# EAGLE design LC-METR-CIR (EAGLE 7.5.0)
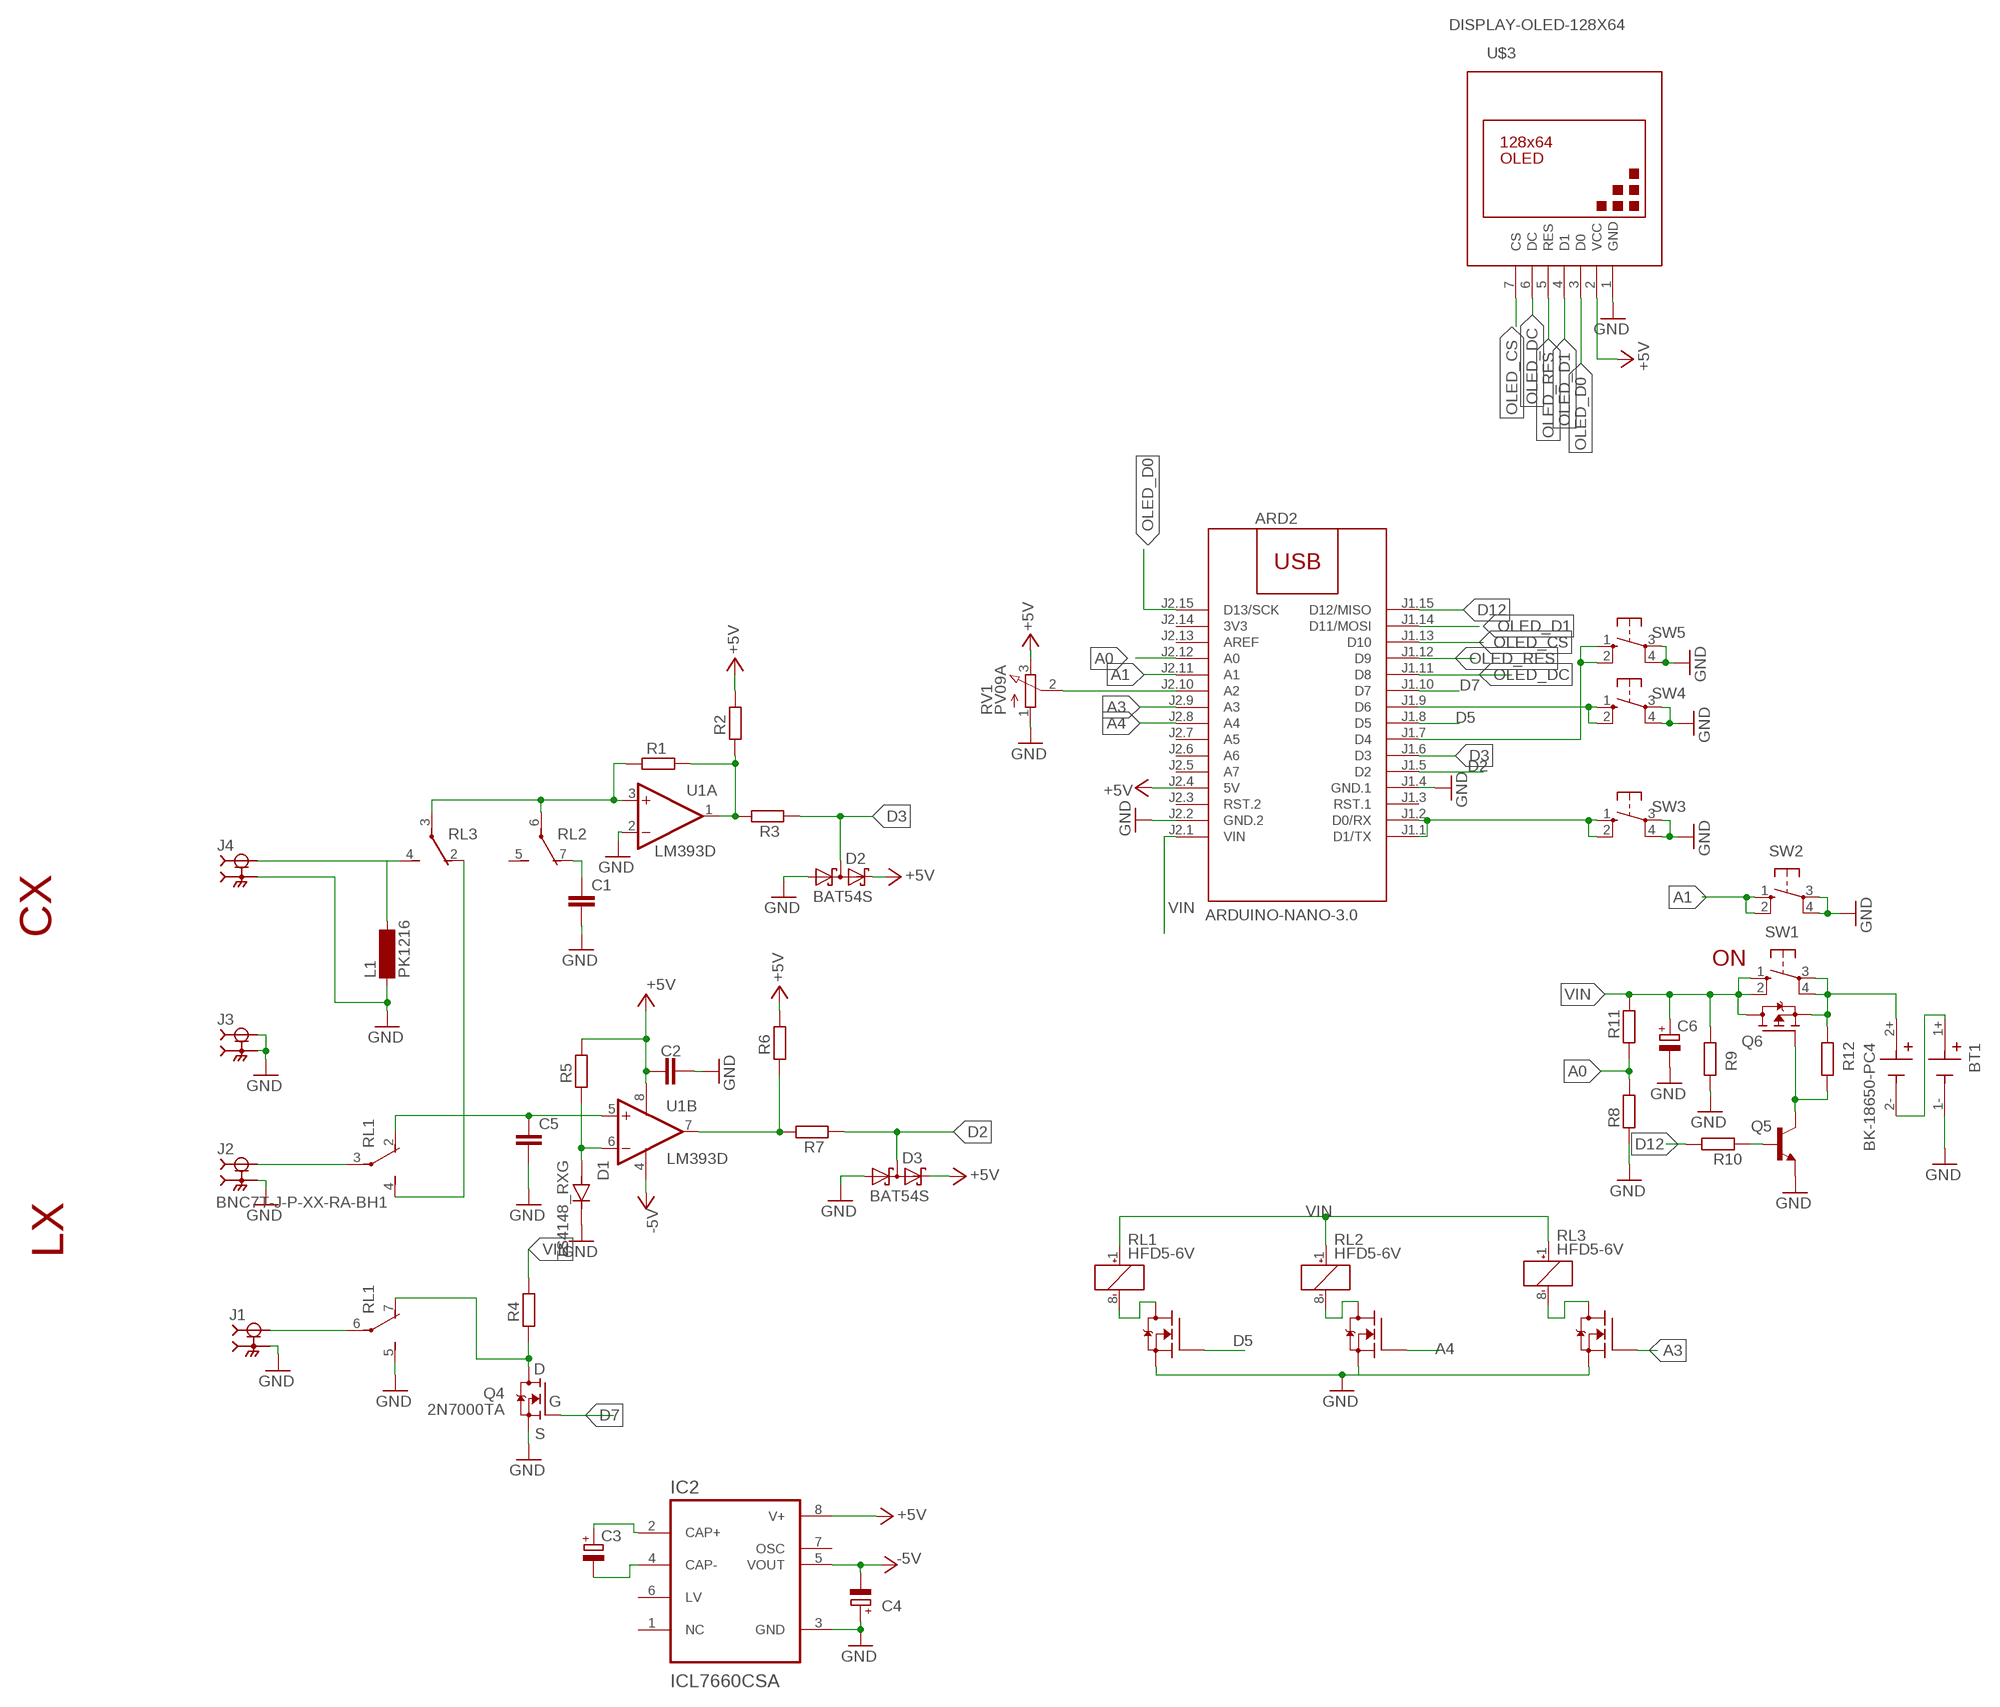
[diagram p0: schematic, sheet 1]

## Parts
ARD2  ARDUINO-NANO-3.0  [ARDUINO-NANO-3.0]
BT1  BK-18650-PC4  [BAT_BK-18650-PC4]
C1  C-EUC1206  [C1206]
C2  C-EUC0805  [C0805]
C3  CPOL-EUSMCA  [SMC_A]
C4  CPOL-EUSMCA  [SMC_A]
C5  C-EUC1206  [C1206]
C6  CPOL-EUSMCA  [SMC_A]
D1  TS4148_RXG  [DIO_TS4148_RXG]
D2  BAT54S  [SOT23]
D3  BAT54S  [SOT23]
IC2  ICL7660CSA  [SOIC127P600X175-8N]
J1  BNC7T-J-P-XX-RA-BH1  [SAMTEC_BNC7T-J-P-XX-RA-BH1]
J2  BNC7T-J-P-XX-RA-BH1  [SAMTEC_BNC7T-J-P-XX-RA-BH1]
J3  BNC7T-J-P-XX-RA-BH1  [SAMTEC_BNC7T-J-P-XX-RA-BH1]
J4  BNC7T-J-P-XX-RA-BH1  [SAMTEC_BNC7T-J-P-XX-RA-BH1]
L1  PK1216  BS11  [BS11]
Q1  ZVN3310F  [SOT23]
Q2  ZVN3310F  [SOT23]
Q3  ZVN3310F  [SOT23]
Q4  2N7000TA  [TO-92]
Q5  BC817-16LT1SMD  [SOT23-BEC]
Q6  STR2P3LLH6  [SOT23]
R1  R-EU_R0805  [R0805]
R2  R-EU_R0805  [R0805]
R3  R-EU_R0805  [R0805]
R4  R-EU_R0805  [R0805]
R5  R-EU_R0805  [R0805]
R6  R-EU_R0805  [R0805]
R7  R-EU_R0805  [R0805]
R8  R-EU_R0805  [R0805]
R9  R-EU_R0805  [R0805]
R10  R-EU_R0805  [R0805]
R11  R-EU_R0805  [R0805]
R12  R-EU_R0805  [R0805]
RL1  HFD5-6V  G6J-2P-Y  [G6J-2P-Y]
RL2  HFD5-6V  G6J-2P-Y  [G6J-2P-Y]
RL3  HFD5-6V  G6J-2P-Y  [G6J-2P-Y]
RV1  PV09A  [PTV09]
SW1  10-XX  [B3F-10XX]
SW2  10-XX  [B3F-10XX]
SW3  10-XX  [B3F-10XX]
SW4  10-XX  [B3F-10XX]
SW5  10-XX  [B3F-10XX]
U1  LM393D  [SO08]
U$3  DISPLAY-OLED-128X64  [DISPLAY-OLED-128X64]

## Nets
+5V: ARD2.J2.4(5V) C2.1 D2.2(C2) D3.2(C2) IC2.8(V+) R2.2 R5.2 R6.2 RV1.3(E) U1.8(P:V+) U$3.2(VCC)
-5V: C4.- IC2.5(VOUT) U1.4(P:V-)
A0: ARD2.J2.12(A0) R8.2 R11.1
A1: ARD2.J2.11(A1) SW2.1(S) SW2.2(S1)
A3: ARD2.J2.9(A3) Q1.2(G)
A4: ARD2.J2.8(A4) Q2.2(G)
BAT: BT1.2+ Q6.3(S) R12.2 SW1.3(P) SW1.4(P1)
D2: ARD2.J1.5(D2) D3.3(C1A2) R7.1
D3: ARD2.J1.6(D3) D2.3(C1A2) R3.1
D5: ARD2.J1.8(D5) Q3.2(G)
D7: ARD2.J1.10(D7) Q4.2(G)
D12: ARD2.J1.15(D12/MISO) R10.2
GND: ARD2.J1.4(GND.1) ARD2.J2.2(GND.2) BT1.1- C1.2 C2.2 C4.+ C5.2 C6.- D1.C(K) D2.1(A1) D3.1(A1) IC2.3(GND) J1.S1 J1.S2 J1.S3 J1.S4 J2.S1 J2.S2 J2.S3 J2.S4 J3.1 J3.S1 J3.S2 J3.S3 J3.S4 J4.S1 J4.S2 J4.S3 J4.S4 L1.1 Q1.3(S) Q2.3(S) Q3.3(S) Q4.1(S) Q5.E R8.1 R9.1 RL1.5(3:S) RV1.1(A) SW2.3(P) SW2.4(P1) SW3.3(P) SW3.4(P1) SW4.3(P) SW4.4(P1) SW5.3(P) SW5.4(P1) U1.2(A:-IN) U$3.1(GND)
N$1: ARD2.J1.1(D1/TX) ARD2.J1.2(D0/RX) SW3.1(S) SW3.2(S1)
N$2: ARD2.J1.9(D6) SW4.1(S) SW4.2(S1)
N$3: R1.1 RL2.6(3:P) RL3.3(2:P) U1.3(A:+IN)
N$4: R1.2 R2.1 R3.2 U1.1(A:OUT)
N$5: ARD2.J1.7(D4) SW5.1(S) SW5.2(S1)
N$6: C3.+ IC2.2(CAP+)
N$7: ARD2.J2.10(A2) RV1.2(S)
N$8: C3.- IC2.4(CAP-)
N$9: R6.1 R7.2 U1.7(B:OUT)
N$10: C1.1 RL2.7(3:O)
N$11: J4.1 L1.2 RL3.4(2:S)
N$12: C5.1 RL1.2(2:O) U1.5(B:+IN)
N$13: RL1.4(2:S) RL3.2(2:O)
N$14: Q4.3(D) R4.1 RL1.7(3:O)
N$15: J2.1 RL1.3(2:P)
N$16: Q5.C Q6.2(G) R12.1
N$17: J1.1 RL1.6(3:P)
N$18: Q5.B R10.1
N$19: Q3.1(D) RL1.8(1:-)
N$20: Q2.1(D) RL2.8(1:-)
N$21: Q1.1(D) RL3.8(1:-)
N$22: BT1.1+ BT1.2-
N$23: D1.A R5.1 U1.6(B:-IN)
OLED_CS: ARD2.J1.13(D10) U$3.7(CS)
OLED_D0: ARD2.J2.15(D13/SCK) U$3.3(D0)
OLED_D1: ARD2.J1.14(D11/MOSI) U$3.4(D1)
OLED_DC: ARD2.J1.11(D8) U$3.6(DC)
OLED_RES: ARD2.J1.12(D9) U$3.5(RES)
VIN: ARD2.J2.1(VIN) C6.+ Q6.1(D) R4.2 R9.2 R11.2 RL1.1(1:+) RL2.1(1:+) RL3.1(1:+) SW1.1(S) SW1.2(S1)
Unconnected: ARD2.J1.3(RST.1) ARD2.J2.3(RST.2) ARD2.J2.5(A7) ARD2.J2.6(A6) ARD2.J2.7(A5) ARD2.J2.13(AREF) IC2.1(NC) IC2.6(LV) IC2.7(OSC) RL2.2(2:O) RL2.3(2:P) RL2.4(2:S) RL2.5(3:S) RL3.5(3:S) RL3.6(3:P) RL3.7(3:O)

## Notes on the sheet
- CX
- ON
- LX

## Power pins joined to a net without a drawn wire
3V3: ARD2.J2.14(3V3)

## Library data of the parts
ARD2 = diy-modules:ARDUINO-NANO-3.0: Arduino Nano 3.0 and compatible devices More details available here: https://www.arduino.cc/en/Main/ArduinoBoardNano Click here to find device on ebay.com
BT1 = BK-18650-PC4:BK-18650-PC4: Battery Holder (Open) 18650 2 Cell PC Pin Check availability; AVAILABILITY: In Stock; CHECK_PRICES: https://www.snapeda.com/parts/BK-18650-PC4/Memory+Protection+Devices/view-part/?ref=eda; DESCRIPTION: Battery Holder (Open) 18650 2 Cell PC Pin; MF: MPD (Memory Protection Devices); MP: BK-18650-PC4; PACKAGE: None; PRICE: None; SNAPEDA_LINK: https://www.snapeda.com/parts/BK-18650-PC4/Memory+Protection+Devices/view-part/?ref=snap
C1 C2 C5 = rcl:C-EU: CAPACITOR, European symbol
C3 C4 C6 = rcl:CPOL-EU: POLARIZED CAPACITOR, European symbol
D1 = TS4148_RXG:TS4148_RXG: Check availability Check availability Check availability; AVAILABILITY: In Stock; CHECK_PRICES: https://www.snapeda.com/parts/TS4148%20RXG/Taiwan+Semiconductor/view-part/?ref=eda; DESCRIPTION: 1206 (Ceramics) 75V 0.15A Switching Diode & Array; MF: Taiwan Semiconductor; MP: TS4148 RXG; PACKAGE: 1206-2 Taiwan Semiconductor; PRICE: None; SNAPEDA_LINK: https://www.snapeda.com/parts/TS4148%20RXG/Taiwan+Semiconductor/view-part/?ref=snap
D2 D3 = diode:BAT54S: Schottky Diodes Pin connection corrected 2011-05-04 Source: Fairchild .. BAT54.pdf
IC2 = ICL7660CSA:ICL7660CSA: Check availability; AVAILABILITY: In Stock; CHECK_PRICES: https://www.snapeda.com/parts/ICL7660CSA/Analog+Devices/view-part/?ref=eda; DESCRIPTION: Charge Pump Switching Regulator IC Positive or Negative Fixed -Vin, nVin, Vin/2 1 Output 20mA 8-SOIC (0.154, 3.90mm Width); MF: Analog Devices; MP: ICL7660CSA; PACKAGE: SOIC-8 Maxim; PRICE: None; SNAPEDA_LINK: https://www.snapeda.com/parts/ICL7660CSA/Analog+Devices/view-part/?ref=snap
J1-J4 = BNC7T-J-P-XX-RA-BH1:BNC7T-J-P-XX-RA-BH1: TRUE 75 OHM RIGHT ANGLE JACK ASSEMBLY Check availability; AVAILABILITY: In Stock; CHECK_PRICES: https://www.snapeda.com/parts/BNC7T-J-P-HN-RA-BH1/Samtec+Inc./view-part/?ref=eda; DESCRIPTION: BNC Connector Jack, Female Socket 75 Ohms Panel Mount, Through Hole, Right Angle Solder; MF: Samtec; MP: BNC7T-J-P-HN-RA-BH1; PACKAGE: None; PRICE: None; PURCHASE-URL: https://www.snapeda.com/api/url_track_click_mouser/?unipart_id=608953&manufacturer=Samtec&part_name=BNC7T-J-P-HN-RA-BH1&search_term=bnc connector; SNAPEDA_LINK: https://www.snapeda.com/parts/BNC7T-J-P-HN-RA-BH1/Samtec+Inc./view-part/?ref=snap
L1 = inductor-neosid:BS: INDUCTOR; OC_FARNELL: unknown; OC_NEWARK: unknown
Q1-Q3 = transistor-fet:ZVN3310F
Q4 = 2N7000TA:2N7000TA: http://www.mouser.com/ds/2/149/2N7000TA-347571.pdf Check availability; AVAILABILITY: In Stock; CHECK_PRICES: https://www.snapeda.com/parts/2N7000-TA/Onsemi/view-part/?ref=eda; DESCRIPTION: N-Channel 60 V 200mA (Tc) 400mW (Ta) Through Hole TO-92-3; MF: ON Semiconductor; MP: 2N7000-TA; PACKAGE: E-PKG AXIAL-LEADED-2 ON Semiconductor; PRICE: None; SNAPEDA_LINK: https://www.snapeda.com/parts/2N7000-TA/Onsemi/view-part/?ref=snap
Q5 = transistor-npn:BC817*: NPN Transistor
Q6 = transistor-fet:STR2P3LLH6
R1-R12 = rcl:R-EU_: RESISTOR, European symbol
RL1-RL3 = relay:G6J*-2?-Y: Surface-Mounting Signal Relay - G6J-Y 5.7 x 10.6 x 9 mm Source: http://www.omroncomponents.eu/ .. K125-E2-02-X.pdf; MF: OMRON COMPONENTS USA; MPN: G6J-2P-Y-DC12; OC_FARNELL: unknown; OC_NEWARK: 70J9830
RV1 = pot:PV09A
SW1-SW5 = switch-omron:10-XX: OMRON SWITCH; MPN: B3F-1000; OC_FARNELL: 176432; OC_NEWARK: 36M3542
U1 = linear:LM393: COMPARATOR
U$3 = diy-modules:DISPLAY-OLED-128X64: 128x64 Dot Matrix OLED Module based on SSD1306 chip Variant with SPI interface More details available here: http://www.instructables.com/id/How-to-use-OLED-display-arduino-module/ SSD1306 datasheet: https://cdn-shop.adafruit.com/datasheets/SSD1306.pdf Click here to find device on ebay.com Note: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

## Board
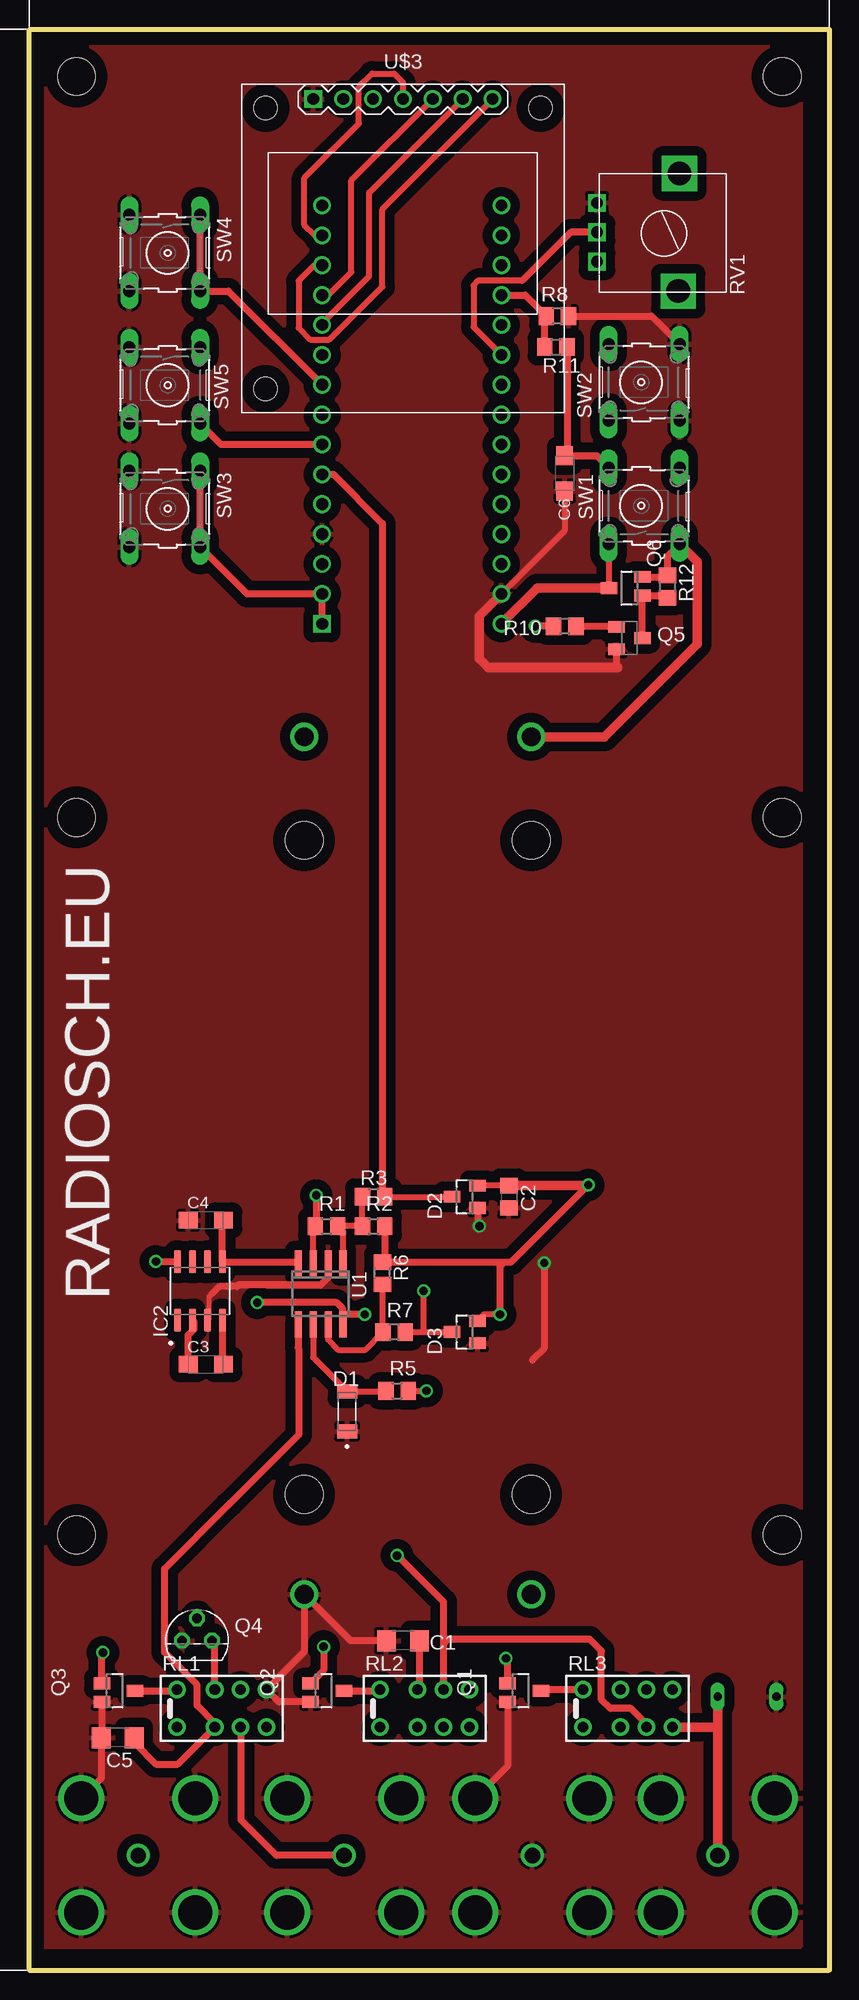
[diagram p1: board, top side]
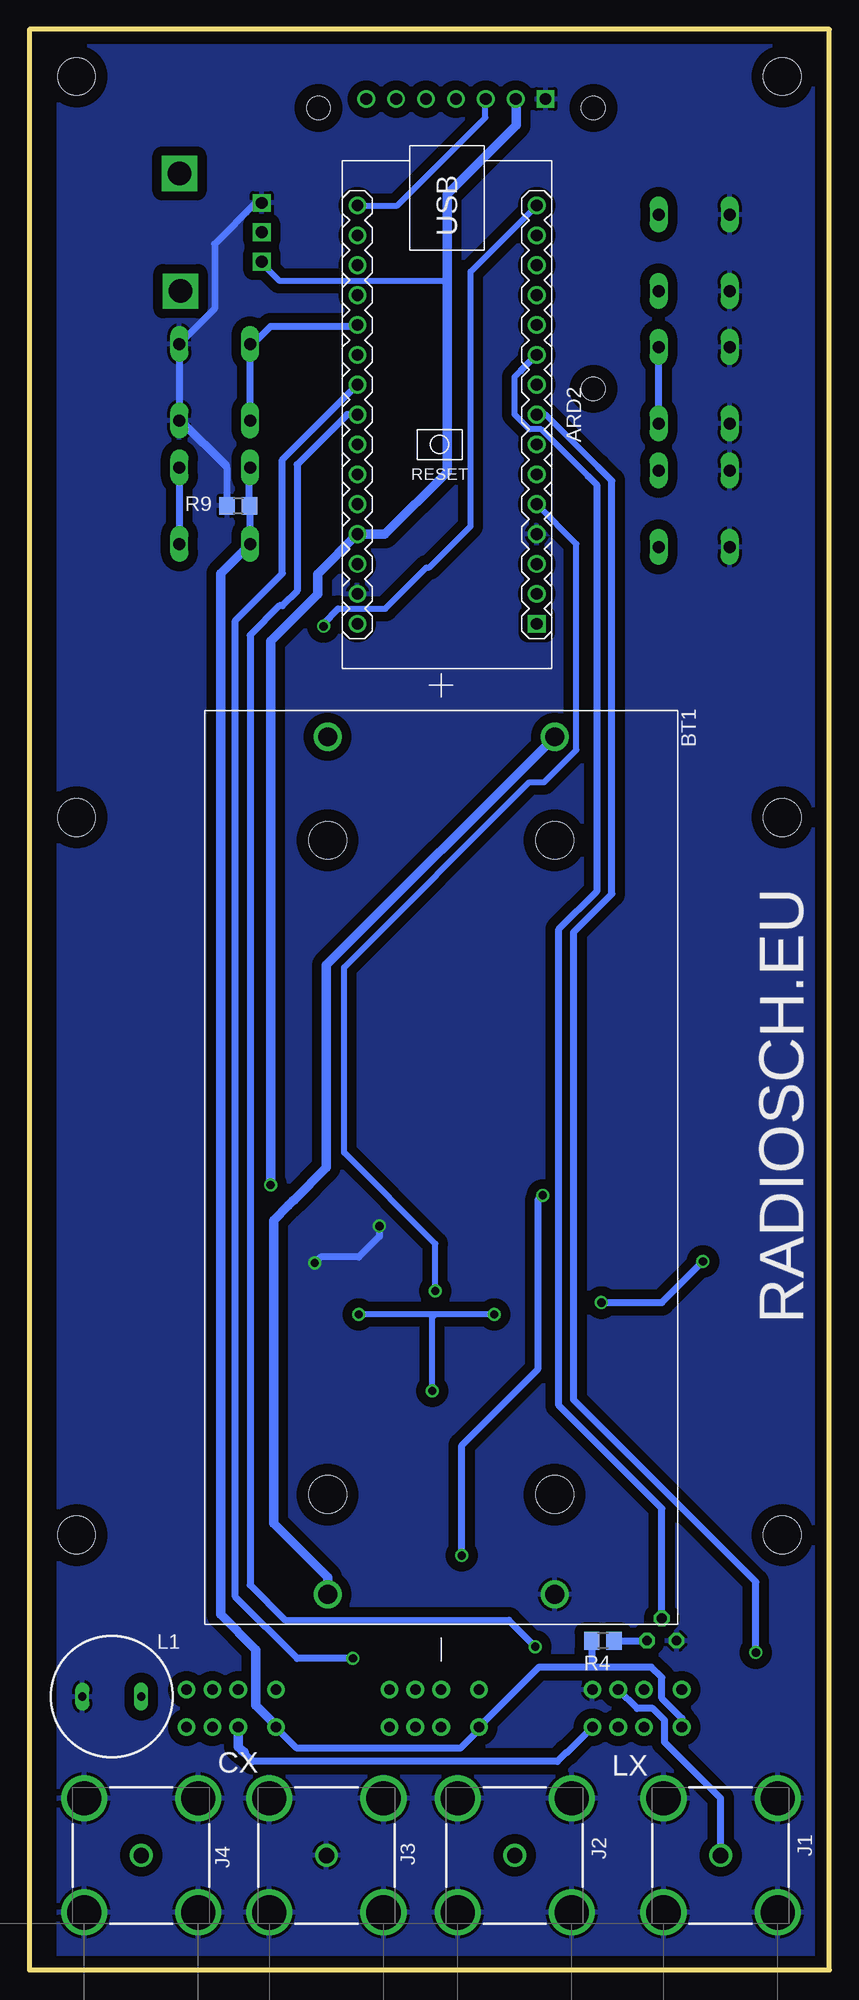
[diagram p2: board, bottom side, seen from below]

Size 68 x 165 mm. Coordinates in mm from the lower left corner, seen from the top.
Outline: 0,0 0,165 68,165 68,0 0,0
Copper layers (1*16): Top 0.035mm / dielectric 1.5mm / Bottom 0.035mm
Design rules "default *": minimum track width 10mil, minimum drill 15mil, track to track 6mil, track to pad 6mil, pad to pad 6mil, via to via 6mil, smd to smd 4mil, copper to edge 40mil, drill to drill 8mil, minimum pad ring 10mil, minimum via ring 8mil, stop-mask expansion 4mil, vias tented up to drill 0mil, thermal gap 10mil
Holes 3.2 mm at 4,161 64,161 4,98 64,98 4,37 64,37

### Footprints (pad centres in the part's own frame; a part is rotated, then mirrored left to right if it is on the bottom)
ARDUINO-NANO-3.0 = drill 1 square: J1.1 17.78,7.62 | drill 1: J1.2 15.24,7.62; J1.3 12.7,7.62; J1.4 10.16,7.62; J1.5 7.62,7.62; J1.6 5.08,7.62; J1.7 2.54,7.62; J1.8 0,7.62; J1.9 -2.54,7.62; J1.10 -5.08,7.62; J1.11 -7.62,7.62; J1.12 -10.16,7.62; J1.13 -12.7,7.62; J1.14 -15.24,7.62; J1.15 -17.78,7.62; J2.1 17.78,-7.62; J2.2 15.24,-7.62; J2.3 12.7,-7.62; J2.4 10.16,-7.62; J2.5 7.62,-7.62; J2.6 5.08,-7.62; J2.7 2.54,-7.62; J2.8 0,-7.62; J2.9 -2.54,-7.62; J2.10 -5.08,-7.62; J2.11 -7.62,-7.62; J2.12 -10.16,-7.62; J2.13 -12.7,-7.62; J2.14 -15.24,-7.62; J2.15 -17.78,-7.62
BAT_BK-18650-PC4 = drill 1.6: 1+ -36.6,9.65; 1- 36.3,9.65; 2+ -36.6,-9.65; 2- 36.3,-9.65 | hole 3.2: -27.81,-9.65; -27.81,9.65; 27.81,-9.65; 27.81,9.65
C1206 = smd 1.6 x 1.8: 1 -1.4,0; 2 1.4,0
C0805 = smd 1.3 x 1.5: 1 -0.95,0; 2 0.95,0
SMC_A = smd 1.6 x 1.4: + -1.5,0; - 1.5,0
DIO_TS4148_RXG = smd 1.2 x 1.7: A 1.7,0; C -1.7,0
SOT23 = smd 1 x 1.4: 1 -0.95,-1.1; 2 0.95,-1.1; 3 0,1.1
SOIC127P600X175-8N = smd 1.97 x 0.59: 1 -2.475,1.905; 2 -2.475,0.635; 3 -2.475,-0.635; 4 -2.475,-1.905; 5 2.475,-1.905; 6 2.475,-0.635; 7 2.475,0.635; 8 2.475,1.905
SAMTEC_BNC7T-J-P-XX-RA-BH1 = drill 1.3: 1 0,0 | drill 2.9: S1 -4.85,4.85; S2 4.85,4.85; S3 4.85,-4.85; S4 -4.85,-4.85
BS11 = drill 0.7 long: 1 -2.5,0; 2 2.5,0
SOT23' = smd 1 x 1.4: 1 0,1.735; 2 -0.632,-1.1; 3 0.95,-1.1
TO-92 = drill 0.813 octagon: 1 -1.27,0; 2 0,1.905; 3 1.27,0
SOT23-BEC = smd 1 x 1.4: B -0.95,-1.1; C 0,1.1; E 0.95,-1.1
R0805 = smd 1.3 x 1.5: 1 -0.95,0; 2 0.95,0
G6J-2P-Y = drill 0.9 pad 1.5: 1 -3.2,-1.6; 2 0,-1.6; 3 2.2,-1.6; 4 4.4,-1.6; 5 4.4,1.6; 6 2.2,1.6; 7 0,1.6; 8 -3.2,1.6
PTV09 = drill 1 square: 1 -2.5,0; 2 0,0; 3 2.5,0 | drill 2 square: P$4 -5,7; P$5 5,6.9
B3F-10XX = drill 1.016 long: 1 -3.251,2.761; 2 3.251,2.761; 3 -3.251,-3.261; 4 3.251,-3.261
SO08 = smd 0.6 x 2.2: 1 -1.905,-2.6; 2 -0.635,-2.6; 3 0.635,-2.6; 4 1.905,-2.6; 5 1.905,2.6; 6 0.635,2.6; 7 -0.635,2.6; 8 -1.905,2.6
DISPLAY-OLED-128X64 = drill 1 square: 1 -7.62,12.7 | drill 1: 2 -5.08,12.7; 3 -2.54,12.7; 4 0,12.7; 5 2.54,12.7; 6 5.08,12.7; 7 7.62,12.7 | hole 2: -11.684,11.938; 11.684,11.938; -11.684,-11.938

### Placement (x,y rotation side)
ARD2  32.5,132.25 270 bottom
BT1  33,68.25 270 bottom
C1  31.75,28 180 top
C2  40.75,65.75 270 top
C3  15,51.5 0 top
C4  15,63.75 0 top
C5  7.5,19.75 180 top
C6  45.5,127.25 270 top
D1  27,47.5 90 top
D2  37,65.75 90 top
D3  37,54.25 90 top
IC2  14.5,57.75 90 top
J1  9.25,9.75 180 bottom
J2  26.75,9.75 180 bottom
J3  42.75,9.75 180 bottom
J4  58.5,9.75 180 bottom
L1  61,23.25 0 bottom
Q1  ZVN3310F  [SOT23']  41.75,23.75 270 top
Q2  ZVN3310F  [SOT23']  25,23.75 270 top
Q3  ZVN3310F  [SOT23']  7.25,23.75 270 top
Q4  14.25,28 0 top
Q5  51,113.25 270 top
Q6  STR2P3LLH6  [SOT23']  51,117.5 90 top
R1  25.25,63.25 0 top
R2  29.25,63.25 0 top
R3  29.25,65.75 180 top
R4  19.25,28 180 bottom
R5  31.25,49.25 0 top
R6  30,59.25 90 top
R7  31,54.25 180 top
R8  44.88,140.62 180 top
R9  50.25,124.5 0 bottom
R10  45.5,114.25 180 top
R11  44.75,138 0 top
R12  54.25,117.62 90 top
RL1  15.75,22.25 0 top
RL2  33,22.25 0 top
RL3  50.25,22.25 0 top
RV1  48.25,147.75 270 top
SW1  52,124.5 90 top
SW2  52,135 90 top
SW3  11.75,124.25 270 top
SW4  11.75,146 270 top
SW5  11.75,134.75 270 top
U1  24.75,57.5 180 top
U$3  31.75,146.38 0 top

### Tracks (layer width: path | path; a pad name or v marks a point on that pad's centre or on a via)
+5V  (via drill 0.7)
  Top 0.51: C2.1 D2.2 | v40,55.75 38.65,55.75 D3.2 | R5.2 v33.75,49.25
  Top 0.61: 40.38,60.2 R6.2 30.2,60.4 R2.2 | 40.38,60.2 40.95,60.2 v47.5,66.75 | v40,55.75 40,59.83 40.38,60.2 | U1.8 26.66,54.97 26.62,55 26.62,55.5 | 26.62,55.5 26.62,56.25 26.12,56.75 v19.38,56.75 | v10.75,60.25 12.57,60.25 IC2.8 | v28.5,55.75 26.88,55.75 26.62,55.5
  Top 0.813: C2.1 47.45,66.7 v47.5,66.75
  Bottom 0.51: RV1.3 48.25,145.12 46.75,143.62 32.88,143.62 32.5,143.25 | v28.5,55.75 33.5,55.75 | 33.5,55.75 v40,55.75 | v33.75,49.25 33.75,55.5 33.5,55.75
  Bottom 0.61: v19.38,56.75 14.25,56.75 v10.75,60.25
  Bottom 0.813: U$3.2 26.62,159.03 26.62,156.88 32.5,151 32.5,143.25 32.5,127.38 37.78,122.09 ARD2.J2.4 43.5,118.71 43.5,117 47.5,113 v47.5,66.75
-5V
  Top 0.61: U1.4 22.72,60.23 IC2.5 16.41,63.66 C4.-
A0
  Top 0.61: ARD2.J2.12 42.14,142.41 R8.2 43.8,140.5 R11.1
A1
  Bottom 0.61: ARD2.J2.11 40.24,139.75 47.5,139.75 49,138.25 SW2.2 SW2.1
A3  (via drill 0.7)
  Top 0.61: Q1.2 40.65,26.35 v40.5,26.5
  Bottom 0.61: v40.5,26.5 45.25,26.5 50.5,31.75 50.5,114.75 46.5,118.75 46.5,128.41 ARD2.J2.9
A4  (via drill 0.7)
  Top 0.61: v25,27.5 25,25.48 Q2.2
  Bottom 0.61: ARD2.J2.8 41,132.25 45.25,128 45.25,117.25 46.5,116 46.75,116 49.25,113.5 49.25,32.75 46.25,29.75 27.25,29.75 v25,27.5
BAT
  Top 0.61: SW1.3 54.25,120.24 R12.2 54.12,118.45 Q6.3
  Top 0.813: BT1.2+ 48.85,104.85 56.75,112.75 56.75,119.76 SW1.3
  Bottom 0.61: SW1.4 SW1.3
D2  (via drill 0.7)
  Top 0.51: 33.5,54.25 D3.3 | R7.1 33.5,54.25 | 33.5,54.25 v33.5,57.75
  Bottom 0.51: v33.5,57.75 33.5,61.75 41.25,69.5 41.25,85.25 25.5,101 24.25,101 21.5,103.75 21.5,121.25 ARD2.J1.5
D3
  Top 0.51: R3.1 D2.3
  Top 0.61: ARD2.J1.6 25.83,127.17 30,123 30,65.95 R3.1
D5  (via drill 0.7)
  Top 0.61: Q3.2 6.15,26.9 v6.25,27
  Bottom 0.51: 19.5,127.62 19.69,127.81 24.12,132.25 ARD2.J1.8
  Bottom 0.61: v6.25,27 6.25,33 21.75,48.5 21.75,88.25 18.5,91.5 18.5,126.62 19.69,127.81 | ARD2.J1.8 24.75,132.25
D7
  Bottom 0.51: 20.5,127 24.5,131 25.5,131 26.75,132.25 26.75,135.46 26.23,135.98
  Bottom 0.61: Q4.2 14.25,39.25 23,48 23,88.5 19.75,91.75 19.75,126.25 20.5,127 | 26.23,135.98 ARD2.J1.10
D12  (via drill 0.7)
  Top 0.61: R10.2 v43,114.25
  Bottom 0.51: 41.75,115.75 37.75,115.75 34.25,119.25 34,119.25 30.5,122.75 30.5,144.41 ARD2.J1.15
  Bottom 0.61: v43,114.25 43,114.5 41.75,115.75
GND  (via drill 0.7)
  Top 0.406: 15.5,57.5 15.25,57.25 15.25,55.39 IC2.3
  Top 0.51: C6.- 45.5,122.39 ARD2.J2.2
  Top 0.61: R8.1 52.89,140.62 SW2.4 | Q5.E 49.9,110.85 50,110.75 | Q3.3 6.15,19.8 C5.2 6.1,16.3 J1.S4 | Q2.3 21.2,22.8 RL1.5 23.35,27.05 BT1.1- 27.3,28 C1.2 | Q1.3 40.65,17.35 J3.S4 | D2.1 38.1,63.4 v38.25,63.25 | v43.75,60.12 43.75,52.88 42.75,51.88 | U1.2 25.39,58.88 24.75,58.25 17.75,58.25 17.62,58.12 16.12,58.12 15.5,57.5
  Top 0.813: 50,110.75 39,110.75 38.25,111.5 38.25,115.14 ARD2.J2.2
  Bottom 0.51: R9.1 51.2,127.95 55,131.75
  Bottom 0.61: R9.1 51.2,127.69 SW2.3 SW2.4 52.25,141.26 52.25,146.75 48.75,150.25 RV1.1 | v38.25,63.25 38.25,62.38 40,60.62 43.25,60.62 v43.75,60.12
  pour Bottom (isolate 0.813): 1,163.62 65.5,163.62 65.5,0.88 1,0.88
  pour Top (isolate 0.813): 0.75,163.5 65.5,163.5 65.5,2 0.75,2
N$1
  Top 0.61: SW3.1 SW3.2 18.5,117.01 ARD2.J1.2 ARD2.J1.1
N$2
  Top 0.61: SW4.1 SW4.2 16.92,142.75 ARD2.J1.9
N$3  (via drill 0.7)
  Top 0.51: U1.3 24.11,63.06 R1.1
  Top 0.61: RL3.3 52.45,20.92 51.12,22.25 49.38,22.25 48.62,23 48.62,27.12 47.62,28.12 35.58,28.12 35.2,27.75 | v24.38,65.88 24.38,63.33 R1.1 | RL2.6 35.2,27.75 | 35.2,27.75 35.2,31.3 v31.25,35.25
  Bottom 0.61: v24.38,65.88 24.75,65.5 24.75,51.12 31.25,44.62 v31.25,35.25
N$4
  Top 0.51: U1.1 26.66,62.8 R1.2 R2.1 R3.2
N$5
  Top 0.61: ARD2.J1.7 16.3,129.71 SW5.2
  Bottom 0.61: SW5.2 SW5.1
N$6
  Top 0.61: C3.+ 13.5,54 14,54.5 14,55.14 IC2.2
N$7
  Top 0.51: 42,143.75 41.88,143.62 38.12,143.62 37.75,143.25 37.75,139.7 ARD2.J2.10
  Top 0.61: RV1.2 46,147.75 42,143.75
N$8
  Top 0.61: IC2.4 16.41,51.59 C3.-
N$9
  Top 0.51: R6.1 30.05,58.25 R7.2 28.55,52.75 26.25,52.75 25.39,53.62 U1.7
N$10
  Top 0.61: C1.1 33.15,24 RL2.7
N$11
  Top 0.813: J4.1 58.5,20.88 | 58.5,20.88 L1.2 | RL3.4 58.27,20.65 58.5,20.88
N$12
  Top 0.61: C5.1 8.9,19.35 10.75,17.5 12.6,17.5 RL1.2 15.75,21 14.25,22.5 14.25,24.25 11.5,27 11.5,34.12 16.88,39.5 17.06,39.69 22.88,45.5 22.88,52.88 22.84,52.91 U1.5
N$13
  Bottom 0.61: RL1.4 22.3,18.5 22.38,18.5 23.12,17.75 49,17.75 49.94,18.69
  Bottom 0.813: RL3.2 50.25,19 49.94,18.69 49.75,18.5
N$14
  Top 0.61: RL1.7 15.75,27.77 Q4.3
  Bottom 0.61: R4.1 Q4.3
N$15
  Top 0.61: J2.1 21,9.75 18,12.75 18,20.6 RL1.3
N$16
  Top 0.61: Q5.C Q6.2 54.06,116.87 R12.1
N$17
  Bottom 0.61: J1.1 9.25,14.62 14,19.38 14,21.25 15,22.25 16.35,22.25 RL1.6
N$18
  Top 0.61: R10.1 49.85,114.25 Q5.B
N$19
  Top 0.61: Q3.1 12.45,23.75 RL1.8
N$20
  Top 0.61: Q2.1 29.7,23.75 RL2.8
N$21
  Top 0.61: RL3.8 43.59,23.85 Q1.1
N$22
  Bottom 0.813: BT1.2- 42.65,33.4 47.25,38 47.25,63.75 46,65 45.62,65.38 45.5,65.5 42.75,68.25 42.75,85.45 BT1.1+
N$23
  Top 0.51: U1.6 24.11,52.09 D1.A 30.25,49.2 R5.1
OLED_CS
  Top 0.51: ARD2.J1.13 24.2,144.95 22.88,143.62 22.88,139.62 23.88,138.62 25.5,138.62 30,143.12 30,149.7 U$3.7
OLED_D0
  Bottom 0.51: ARD2.J2.15 36.72,150.03 29.25,157.5 29.25,159.03 U$3.3
OLED_D1
  Top 0.51: U$3.4 31.75,160.5 31,161.25 29.12,161.25 28,160.12 28,157 23.38,152.38 23.38,148.38 24.26,147.49 ARD2.J1.14
OLED_DC
  Top 0.51: ARD2.J1.11 24.88,140 28.88,144 28.88,151.12 U$3.6
OLED_RES
  Top 0.51: ARD2.J1.12 25.41,142.41 27.38,144.38 27.38,152.16 U$3.5
VIN
  Top 0.51: Q6.1 49.27,121.22 SW1.1
  Top 0.61: C6.+ 46,128.75 | 46,128.75 48.24,128.75 SW1.2 | R11.2 45.7,129.05 46,128.75
  Top 0.813: Q6.1 43.15,117.5 ARD2.J2.1
  Bottom 0.61: SW1.2 49.3,127.69 R9.2 49.24,124.44 SW1.1 | RL1.1 12.55,21.42 14.25,23.12 14.25,24.88 15.12,25.75 20,25.75 | 20,25.75 24.7,25.75 RL2.1 29.8,20.45 31.38,18.88 45.27,18.88 RL3.1 | R4.2 20.2,25.95 20,25.75
  Bottom 0.813: RL3.1 47.05,20.8 48.75,22.5 48.75,27.25 51.75,30.25 51.75,118.74 SW1.1

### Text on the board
tPlace: RADIOSCH.EU
bPlace: RADIOSCH.EU | CX | LX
